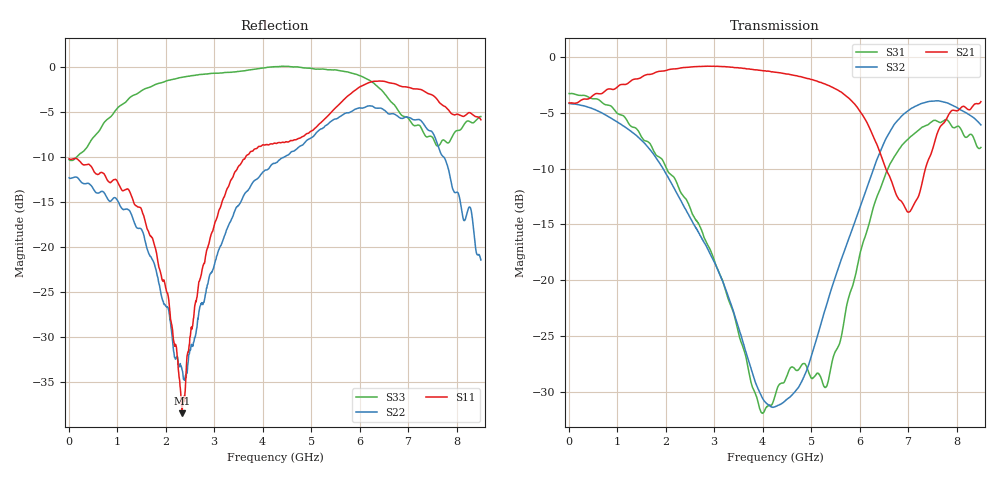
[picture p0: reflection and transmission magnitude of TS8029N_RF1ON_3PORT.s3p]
!Created with skrf (http://scikit-rf.org).
# GHz S RI R 50.0
!freq ReS11 ImS11 ReS12 ImS12 ReS13 ImS13
! ReS21 ImS21 ReS22 ImS22 ReS23 ImS23
! ReS31 ImS31 ReS32 ImS32 ReS33 ImS33
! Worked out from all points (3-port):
!   1601 points, 10 MHz to 8.5 GHz, reference 50 ohm
!   strongest paths, dB at 10 MHz, 2.132 GHz, 4.255 GHz, 6.378 GHz, 8.5 GHz:
!     S21: -4.1, -1.1, -1.4, -8.1, -4.0
!     S32: -4.2, -11.4, -31.3, -9.0, -6.1
!     S31: -3.3, -10.6, -30.4, -12.3, -8.1
!   lowest |S11| = -38.4 dB at 2.339 GHz (marker M1), VSWR 1.02, Z = 48.8 + j0.142 ohm
!   |S11| at or under -10 dB: start of sweep to 3.645 GHz
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0.01  -0.3107 0.00384  0.6231 -1.11e-05  0.6861 -0.00692
      0.6231 3.75e-05  -0.2436 0.00289  0.619 -0.00747
      0.6861 -0.00694  0.6191 -0.00745  -0.3068 0.0108
0.9969625  -0.1637 0.1684  0.7243 -0.101  0.3179 -0.4621
           0.7245 -0.1012  -0.0841 0.1637  0.2553 -0.4444
           0.3177 -0.462  0.2558 -0.4444  0.3528 0.4731
1.766369  -0.0388 0.0961  0.7698 -0.3546  -0.0211 -0.3746
          0.7697 -0.3546  0.0463 0.0664  -0.1039 -0.3476
          -0.0211 -0.3748  -0.1043 -0.3478  0.7976 -0.0226
2.339444  -0.0119 0.00146  0.6866 -0.5741  -0.113 -0.2142
          0.6865 -0.5742  0.0119 -0.0171  -0.1631 -0.1508
          -0.1131 -0.2145  -0.1633 -0.1505  0.7309 -0.4935
3.1513  -0.122 -0.1241  0.4291 -0.7982  -0.0834 -0.0595
        0.4286 -0.7983  -0.1009 -0.0257  -0.102 -0.00267
        -0.0835 -0.0596  -0.1019 -0.00292  0.1634 -0.9166
4.255  -0.342 -0.1639  -0.039 -0.854  0.00258 -0.0303
       -0.0395 -0.8534  -0.2905 0.0385  0.00991 0.0253
       0.00246 -0.0302  0.0099 0.0253  -0.5996 -0.8107
5.257881  -0.5093 0.0118  -0.3909 -0.6524  -0.0325 -0.009
          -0.3903 -0.6527  -0.211 0.4118  0.0426 0.0559
          -0.0325 -0.00898  0.0427 0.0559  -0.9775 0.0353
6.41995  -0.5449 0.6394  -0.337 -0.1599  0.1588 0.1997
         -0.3369 -0.1607  0.1809 0.5649  0.3675 0.0726
         0.1589 0.1997  0.3673 0.0721  -0.4062 0.6426
7.52365  0.1167 0.6861  -0.0519 -0.3949  0.3538 -0.3793
         -0.052 -0.3953  0.4227 -0.0556  0.1026 -0.6273
         0.355 -0.3794  0.1036 -0.6265  0.2459 0.3148
8.5  0.1779 0.4797  -0.38 -0.5035  -0.1718 -0.3537
     -0.3809 -0.5029  0.077 -0.0361  -0.4184 -0.2663
     -0.1722 -0.3536  -0.4184 -0.2673  0.5256 0.0905
